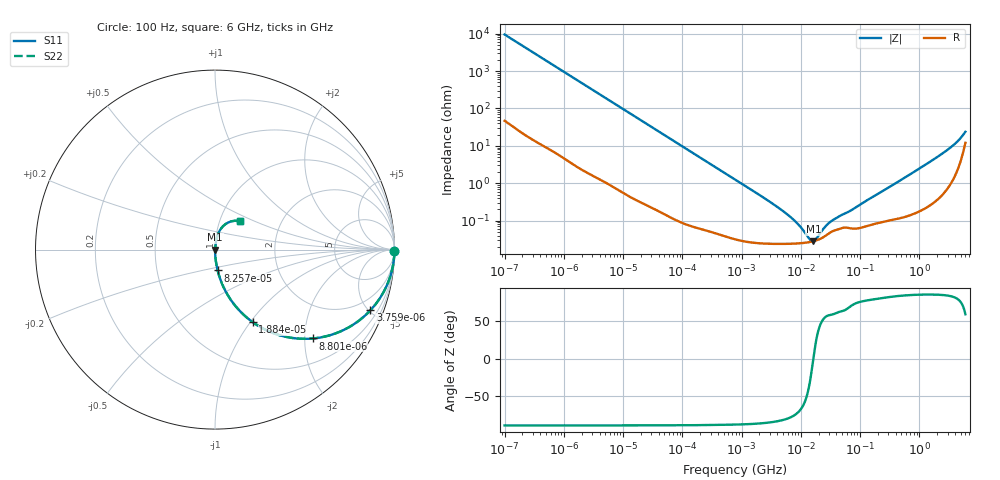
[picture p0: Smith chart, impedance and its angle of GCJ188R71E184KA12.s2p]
!Murata Part Number: GCJ188R71E184KA12
!These Parameters are Measured in Series Mode Connection
!Data Generated on Mar 13, 2026
!  o--ll--o
!Port1  Port2
!  o------o
!Operation Temp=25[degC], DC Bias Voltage=0[V]
!Freq. Start=100[Hz] Stop=6[GHz] 401[Steps]
# Hz S RI R 50
!Freq.(Hz) S11(Real) S11(Imag) S21(Real) S21(Imag) S12(Real) S12(Imag) S22(Real) S22(Imag)
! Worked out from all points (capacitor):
!   401 points, 100 Hz to 6 GHz, reference 50 ohm
!   read as one part in series: C = 167 nF near 109 Hz
!   lowest |Z| = 28.1 mohm at 16.27 MHz (marker M1)
!   series resonance near 16.26 MHz, so ESL is about 570 pH
!   S11 on the Smith chart (normalised r, x): 100 Hz: open; 3.759 kHz: 1.03, -5.12; 8.801 kHz: 1.01, -2.19; 18.84 kHz: 1.01, -1.03; 82.57 kHz: 1.00, -0.24; 6 GHz: 1.24, +0.41
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100  0.9998 -0.0105  0.000162 0.0105  0.000162 0.0105  0.9998 -0.0105
600  0.9958 -0.0624  0.00421 0.0624  0.00421 0.0624  0.9958 -0.0624
2008  0.9572 -0.2  0.0428 0.2  0.0428 0.2  0.9572 -0.2
3759  0.8662 -0.3378  0.1338 0.3378  0.1338 0.3378  0.8662 -0.3378
5625  0.7446 -0.4333  0.2554 0.4333  0.2554 0.4333  0.7446 -0.4333
8801  0.5456 -0.4951  0.4544 0.4951  0.4544 0.4951  0.5456 -0.4951
18841  0.2101 -0.4043  0.7899 0.4043  0.7899 0.4043  0.2101 -0.4043
40335  0.0562 -0.2267  0.9438 0.2267  0.9438 0.2267  0.0562 -0.2267
82567  0.0146 -0.116  0.9854 0.116  0.9854 0.116  0.0146 -0.116
774597  0.000478 -0.0127  0.9995 0.0127  0.9995 0.0127  0.000478 -0.0127
5809218  0.000241 -0.00149  0.9998 0.00149  0.9998 0.00149  0.000241 -0.00149
8692127  0.000246 -0.000813  0.9998 0.000813  0.9998 0.000813  0.000246 -0.000813
1.360128e7  0.000265 -0.000219  0.9997 0.000219  0.9997 0.000219  0.000265 -0.000219
1.555665e7  0.000276 -5.39e-05  0.9997 5.39e-05  0.9997 5.39e-05  0.000276 -5.39e-05
1.626902e7  0.000281 7e-07  0.9997 -7e-07  0.9997 -7e-07  0.000281 7e-07
1.86079e7  0.000299 0.000165  0.9997 -0.000165  0.9997 -0.000165  0.000299 0.000165
2.662322e7  0.000402 0.000607  0.9996 -0.000607  0.9996 -0.000607  0.000402 0.000607
3.330331e7  0.000509 0.000849  0.9995 -0.000849  0.9995 -0.000849  0.000509 0.000849
3.124326e8  0.00106 0.00784  0.9989 -0.00784  0.9989 -0.00784  0.00106 0.00784
2.450438e9  0.00864 0.0613  0.9914 -0.0613  0.9914 -0.0613  0.00864 0.0613
4.385646e9  0.0366 0.1209  0.9634 -0.1209  0.9634 -0.1209  0.0366 0.1209
6e9  0.1365 0.1584  0.8635 -0.1584  0.8635 -0.1584  0.1365 0.1584
